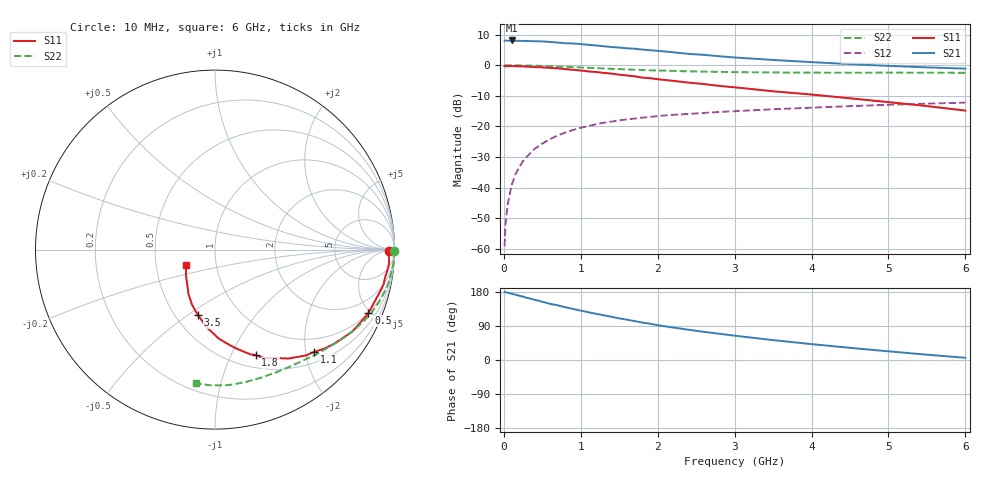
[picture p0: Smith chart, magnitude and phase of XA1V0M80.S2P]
! SIEMENS Discrete & RF Semiconductors
! BFY180
! Si NPN RF Bipolar Junction Transistor in MICRO-X
! VCE = 1 V  IC = 0.8 mA
! Common Emitter S-Parameters:  May  1997
# GHz  S  MA  R  50
!  f  S11  S21  S12  S22
! GHz  MAG  ANG  MAG  ANG  MAG  ANG  MAG  ANG
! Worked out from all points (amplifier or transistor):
!   36 points, 10 MHz to 6 GHz, reference 50 ohm
!   highest |S21| = 8.1 dB at 100 MHz (marker M1)
!   |S21| within 3 dB of that: start of sweep to 1.814 GHz
!   unconditionally stable (mu >= 1): 3.489 GHz to end of sweep
!   at 250 MHz: K = 0.08, MSG = 19.6 dB, |S12| = -31.3 dB
!   at 1.4 GHz: K = 0.53, MSG = 12.2 dB, |S12| = -18.4 dB
!   at 6 GHz: K = 1.10, MAG = 3.6 dB, |S12| = -12.2 dB
!   S11 on the Smith chart (normalised r, x): 10 MHz: 60, -10; 500 MHz: 1.00, -4.85; 1.1 GHz: 0.71, -2.18; 1.8 GHz: 0.64, -1.25; 3.5 GHz: 0.64, -0.55; 6 GHz: 0.71, -0.13
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0.01  0.9682 -0.3  2.529 179.8  0.0011 88.4  0.9977 -0.3
0.02  0.9619 -0.7  2.543 178.9  0.0024 94.2  0.9979 -0.5
0.05  0.9695 -2.2  2.518 177.6  0.0053 87.0  0.9974 -1.4
0.1  0.9728 -4.4  2.55 175.0  0.0108 87.8  0.9966 -2.7
0.15  0.9678 -6.8  2.518 172.4  0.0164 85.1  0.9974 -4.1
0.25  0.9592 -11.5  2.506 167.1  0.0273 82.3  0.9927 -6.8
0.4  0.9363 -17.7  2.474 159.1  0.0429 76.9  0.9845 -10.7
0.5  0.9249 -22.4  2.465 153.7  0.0524 73.9  0.9766 -13.3
0.6  0.9071 -26.4  2.41 148.3  0.0621 71.0  0.966 -15.9
0.9  0.8453 -38.5  2.273 134.7  0.0878 62.2  0.9354 -22.9
1.1  0.7942 -45.8  2.162 126.0  0.1016 57.0  0.9097 -27.2
1.2  0.777 -49.4  2.112 121.8  0.109 54.6  0.9 -29.4
1.5  0.7027 -59.4  1.951 109.9  0.1256 48.7  0.8661 -35.0
1.8  0.6293 -68.9  1.812 98.9  0.1392 43.8  0.8379 -40.0
2  0.5928 -74.0  1.725 91.8  0.1479 40.5  0.823 -43.2
2.2  0.5568 -78.8  1.635 85.8  0.1549 37.5  0.8109 -46.4
2.6  0.494 -87.9  1.482 74.3  0.1665 33.0  0.7884 -51.9
2.8  0.4603 -92.1  1.408 69.3  0.1724 31.0  0.7803 -54.6
3.5  0.3761 -104.8  1.224 52.5  0.1908 24.6  0.7635 -63.8
4.5  0.2885 -120.8  1.046 32.1  0.2147 16.0  0.7572 -77.1
5.5  0.2155 -138.7  0.925 14.0  0.2361 7.7  0.7573 -91.2
6  0.1816 -152.2  0.883 5.8  0.2452 3.3  0.7532 -98.2
